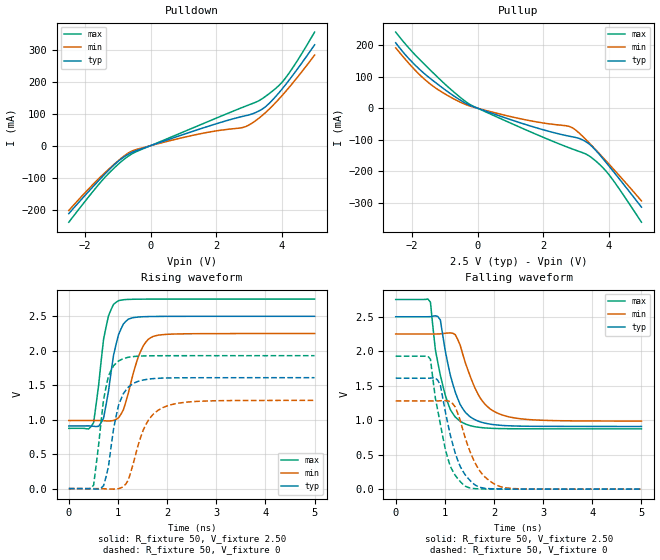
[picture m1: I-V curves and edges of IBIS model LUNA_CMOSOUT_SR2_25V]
[IBIS Ver]   3.2
[Comment Char]   |_char
[File name]   sg8201cga_25v_c.ibs
[File Rev]   1.1
[Date]   2021/10/19 9:35:58
[Source]
[Notes]
[Disclaimer]
This information is for modeling purposes only, and is not guaranteed.
Property of SEIKO EPSON Corp.,
unauthorized reproduction and/or distribution is strictly prohibited.
[Copyright]
Copyright 2021, SEIKO EPSON Corp.
[Component]   2G005_2016
Si_location Pin
Timing_location Pin
[Manufacturer]   SEIKO EPSON Corp.
| 2016 PKG
[Package]
R_pkg   42m   NA   NA
L_pkg   0.49n   NA   NA
C_pkg   0.178p   NA   NA
[Pin] signal_name   model_name
1   OE   NC
2   GND   GND
3   OUT   LUNA_CMOSOUT_SR2_25V
4   VCC   POWER
| Models and submodels in the file (1): LUNA_CMOSOUT_SR2_25V (Output)
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[Model]   LUNA_CMOSOUT_SR2_25V
Model_type Output
Polarity Non-Inverting
Vmeas=1.25
C_comp   2.5p   2.0p   3.0p
[Temperature Range] 25   140   -40
[Voltage Range]   2.50   2.25   2.75
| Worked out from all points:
|   slope of the pulldown table from 0 to 0.375 V, typ, clamps not added: 28.4 ohm
|   slope of the pullup table from 0 to 0.375 V, typ, clamps not added: 27.2 ohm
|   falling waveform, R_fixture 50, V_fixture 2.50: 20-80 % time 344ps typ, 459ps min, 307ps max; typ from 2.5 V to 0.91 V
|   falling waveform, R_fixture 50, V_fixture 0: 20-80 % time 351ps typ, 420ps min, 320ps max; typ from 1.61 V to 0 V
|   rising waveform, R_fixture 50, V_fixture 2.50: 20-80 % time 232ps typ, 313ps min, 206ps max; typ from 0.91 V to 2.5 V
|   rising waveform, R_fixture 50, V_fixture 0: 20-80 % time 248ps typ, 385ps min, 215ps max; typ from 0 V to 1.61 V
[Pullup]
-2.5V     207.5mA    191.6mA    241.6mA
-2V       146.6mA    131.1mA    179.7mA
-1.5V     99.09mA    81.27mA    126.9mA
-1.1V     66.86mA    51.87mA    86.54mA
-500mV    23.87mA    17.83mA    32.02mA
-200mV    7.582mA    5.804mA    9.842mA
1.2V      -42.82mA   -30.98mA   -56.1mA
2.9V      -90.84mA   -62.39mA   -129.6mA
3.4V      -113mA     -109.4mA   -150.9mA
3.9V      -169.4mA   -164.9mA   -197.2mA
4.3V      -221mA     -210.8mA   -252.6mA
5V        -313.8mA   -294mA     -361.5mA
[Pulldown]
-2.5V     -212.6mA   -202.8mA   -239.4mA
-1.9V     -143.9mA   -136mA     -160.7mA
-1.4V     -88.97mA   -84.95mA   -99.42mA
-1V       -49.59mA   -48.07mA   -58.97mA
-600mV    -22.46mA   -18.19mA   -27.32mA
1.3V      45.19mA    32.44mA    55.83mA
2.8V      91.27mA    56.35mA    119.5mA
3.1V      99.17mA    70.8mA     131.5mA
3.5V      121.3mA    103mA      153.7mA
4V        175.9mA    155.6mA    197.2mA
4.4V      228.8mA    204mA      253.7mA
5V        315.1mA    283mA      354.9mA
[Falling Waveform]
R_fixture=50
V_fixture=2.50
V_fixture_min=2.25
V_fixture_max=2.75
0s        2.5V       2.25V      2.75V
707.1ps   2.501V     2.25V      2.711V
808.1ps   2.513V     2.249V     2.018V
909.1ps   2.453V     2.252V     1.651V
1.01ns    2V         2.261V     1.359V
1.212ns   1.407V     2.24V      1.046V
1.364ns   1.168V     1.959V     964.4mV
1.717ns   976.2mV    1.325V     895mV
2.121ns   927mV      1.088V     878.7mV
5ns       909.5mV    987.6mV    874.6mV
[Falling Waveform]
R_fixture=50
V_fixture=0
V_fixture_min=0
V_fixture_max=0
0s        1.609V     1.28V      1.928V
707.1ps   1.61V      1.279V     1.884V
808.1ps   1.613V     1.279V     1.318V
909.1ps   1.51V      1.281V     942mV
1.01ns    1.124V     1.284V     578.4mV
1.212ns   520.9mV    1.192V     199.3mV
1.414ns   207.7mV    744.2mV    43.81mV
1.717ns   26.86mV    258mV      4.171mV
2.121ns   3.292mV    39.41mV    1.348mV
5ns       325.9uV    600.5uV    193.8uV
[Rising Waveform]
R_fixture=50
V_fixture=2.50
V_fixture_min=2.25
V_fixture_max=2.75
0s        909.5mV    987.4mV    874.6mV
505.1ps   904.4mV    987.7mV    959.3mV
656.6ps   954.3mV    986.7mV    1.844V
757.6ps   1.214V     983.3mV    2.345V
909.1ps   1.932V     987.8mV    2.673V
1.01ns    2.231V     1.027V     2.726V
1.111ns   2.389V     1.145V     2.74V
1.414ns   2.489V     1.914V     2.748V
1.717ns   2.497V     2.208V     2.749V
5ns       2.5V       2.25V      2.75V
[Rising Waveform]
R_fixture=50
V_fixture=0
V_fixture_min=0
V_fixture_max=0
0s        0V         0V         0V
505.1ps   -3.54mV    258.4uV    51.53mV
707.1ps   41.46mV    -1.643mV   1.291V
757.6ps   172.4mV    -3.759mV   1.474V
808.1ps   326.4mV    -5.781mV   1.639V
1.01ns    1.206V     -349.9uV   1.851V
1.212ns   1.473V     127.8mV    1.906V
1.566ns   1.582V     925.1mV    1.926V
1.919ns   1.604V     1.177V     1.928V
5ns       1.609V     1.28V      1.928V
[Ramp]
R_load=50
dV/dt_r   9.654E-1/2.478E-10   7.677E-1/3.847E-10   1.157E+0/2.129E-10
dV/dt_f   9.543E-1/3.436E-10   7.574E-1/4.558E-10   1.125E+0/3.071E-10
|[End   LUNA_CMOSOUT_SR2_25V
